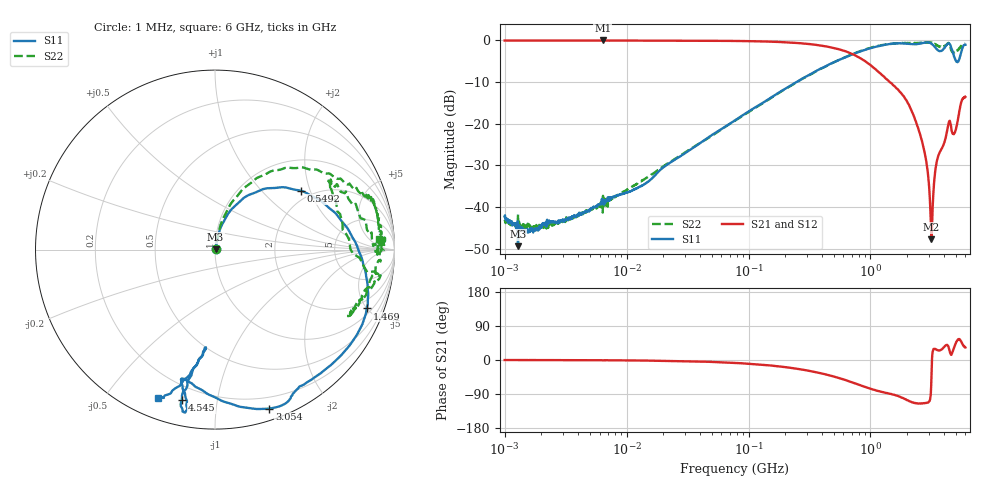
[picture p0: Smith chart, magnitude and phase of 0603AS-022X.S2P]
!s-Parameter Generated by FASTRON Sdn. Bhd.
!FASTRON P/N : 0603AS-022X
!Keysight Technologies: E5071C_MY46733604_B.14.02
!Date: Thu Nov 23 10:35:36 2023
!Version  :Rev01  Thu Nov 23 10:35:36 2023
!Data & Calibration Information:
!Freq  S11:SOLT2(ON)  S21:SOLT2(ON)  S12:SOLT2(ON)  S22:SOLT2(ON)
!PortZ  Port1:50+j0  Port2:50+j0
!When reading reference impedance value at option line is always used.
! Remarks : This data is being provided solely for informational purposes.
# Hz S dB R 50
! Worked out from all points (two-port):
!   1601 points, 1 MHz to 6 GHz, reference 50 ohm
!   highest |S21| = -0.03 dB at 6.378 MHz (marker M1); lowest = -47.7 dB at 3.159 GHz (marker M2)
!   |S21| within 3 dB of the highest: start of sweep to 677.5 MHz
!   lowest |S11| = -49.4 dB at 1.288 MHz (marker M3), VSWR 1.01, Z = 50.3 + j0.108 ohm
!   |S11| at or under -10 dB: start of sweep to 247.9 MHz
!   |S22| runs from -45.6 to -0.4 dB; largest |S21 - S12| = 0.0086
!   S11 on the Smith chart (normalised r, x): 1 MHz: 1.01, +0.01; 549.2 MHz: 1.75, +1.73; 1.469 GHz: 1.35, -4.99; 3.054 GHz: 0.10, -1.39; 4.545 GHz: 0.13, -0.80; 6 GHz: 0.09, -0.68
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1000000  -42.30 19.7  -0.05 -0.1  -0.05 -0.1  -43.07 19.2
1287650  -49.41 18.4  -0.05 -0.1  -0.04 -0.1  -41.77 10.4
4277066  -41.81 53.8  -0.06 -0.5  -0.05 -0.5  -41.73 54.1
6378092  -39.06 66.9  -0.03 -0.8  -0.08 -0.8  -41.34 66.5
1.823719e7  -31.56 75.8  -0.06 -1.9  -0.07 -1.9  -31.06 73.8
7.757876e7  -19.20 76.4  -0.15 -7.6  -0.15 -7.6  -19.26 78.0
3.307917e8  -7.94 53.8  -0.95 -30.0  -0.95 -30.0  -8.02 63.4
5.492243e8  -4.72 34.4  -2.13 -47.4  -2.13 -47.4  -4.71 50.4
8.134906e8  -2.74 11.6  -4.15 -65.9  -4.15 -66.0  -2.67 35.9
1.414819e9  -0.90 -19.2  -9.81 -88.7  -9.83 -88.7  -0.90 18.4
1.468808e9  -0.85 -21.2  -10.20 -89.5  -10.21 -89.5  -0.86 19.4
1.981825e9  -0.80 -43.8  -14.53 -105.5  -14.54 -105.4  -0.68 10.1
2.45304e9  -0.85 -60.4  -20.97 -114.8  -20.95 -114.7  -0.71 2.5
2.848597e9  -0.51 -65.3  -28.50 -113.5  -28.46 -113.5  -0.59 3.3
3.053701e9  -0.57 -71.2  -37.00 -108.1  -36.96 -108.2  -0.57 1.7
3.158731e9  -0.78 -76.0  -47.75 -46.3  -47.77 -46.3  -0.59 -0.7
3.482718e9  -2.09 -95.2  -29.33 27.5  -29.33 27.3  -1.11 -13.7
3.806705e9  -2.55 -104.7  -26.14 27.1  -26.14 27.0  -1.66 -25.7
4.292686e9  -0.80 -100.2  -20.97 38.5  -20.99 38.5  -0.85 -11.4
4.545048e9  -1.33 -102.4  -20.18 15.7  -20.21 15.6  -1.85 -3.3
5.104645e9  -5.14 -96.0  -20.41 50.0  -20.42 50.2  -2.56 29.6
6e9  -1.07 -110.9  -13.59 33.0  -13.59 33.1  -0.77 3.8
